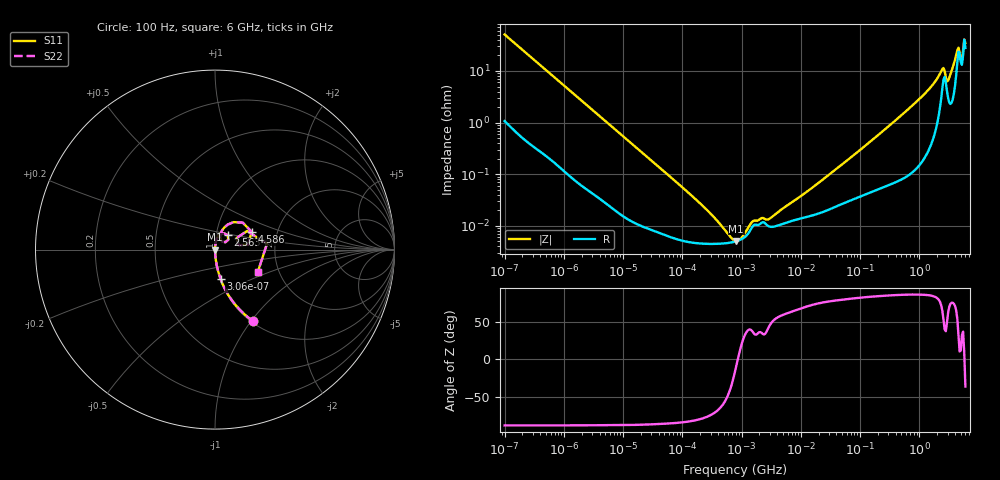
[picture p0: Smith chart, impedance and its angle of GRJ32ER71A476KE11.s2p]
!Murata Part Number: GRJ32ER71A476KE11
!These Parameters are Measured in Series Mode Connection
!Data Generated on Jun 19, 2026
!  o--ll--o
!Port1  Port2
!  o------o
!Operation Temp=25[degC], DC Bias Voltage=0[V]
!Freq. Start=100[Hz] Stop=6[GHz] 401[Steps]
# Hz S RI R 50
!Freq.(Hz) S11(Real) S11(Imag) S21(Real) S21(Imag) S12(Real) S12(Imag) S22(Real) S22(Imag)
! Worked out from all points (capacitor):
!   401 points, 100 Hz to 6 GHz, reference 50 ohm
!   read as one part in series: C = 31 uF near 109 Hz
!   lowest |Z| = 5.06 mohm at 810.1 kHz (marker M1)
!   series resonance near 863.7 kHz, so ESL is about 1.1 nH
!   S11 on the Smith chart (normalised r, x): 100 Hz: 1.02, -1.02; 306 Hz: 1.01, -0.34; 2.563 GHz: 1.14, +0.18; 4.586 GHz: 1.48, +0.31; 6 GHz: 1.56, -0.42
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100  0.2116 -0.3981  0.7884 0.3981  0.7884 0.3981  0.2116 -0.3981
306  0.0308 -0.163  0.9692 0.163  0.9692 0.163  0.0308 -0.163
2008  0.00129 -0.0264  0.9987 0.0264  0.9987 0.0264  0.00129 -0.0264
40335  7.49e-05 -0.00137  0.9999 0.00137  0.9999 0.00137  7.49e-05 -0.00137
184852  4.58e-05 -0.000291  1 0.000291  1 0.000291  4.58e-05 -0.000291
432798  4.49e-05 -9.84e-05  1 9.84e-05  1 9.84e-05  4.49e-05 -9.84e-05
774597  4.92e-05 -1.46e-05  1 1.46e-05  1 1.46e-05  4.92e-05 -1.46e-05
810067  4.99e-05 -8.6e-06  1 8.6e-06  1 8.6e-06  4.99e-05 -8.6e-06
1267578  6.87e-05 5.51e-05  0.9999 -5.51e-05  0.9999 -5.51e-05  6.87e-05 5.51e-05
2169299  0.000114 8.22e-05  0.9999 -8.22e-05  0.9999 -8.22e-05  0.000114 8.22e-05
2967816  9.64e-05 9.74e-05  0.9999 -9.74e-05  0.9999 -9.74e-05  9.64e-05 9.74e-05
1.555665e7  0.000158 0.000522  0.9998 -0.000522  0.9998 -0.000522  0.000158 0.000522
3.124326e8  0.000696 0.00871  0.9993 -0.00871  0.9993 -0.00871  0.000696 0.00871
1.094528e9  0.00268 0.0315  0.9973 -0.0315  0.9973 -0.0315  0.00268 0.0315
2.34314e9  0.037 0.0887  0.963 -0.0887  0.963 -0.0887  0.037 0.0887
2.562649e9  0.0706 0.0797  0.9294 -0.0797  0.9294 -0.0797  0.0706 0.0797
3.065283e9  0.032 0.0543  0.968 -0.0543  0.968 -0.0543  0.032 0.0543
3.666503e9  0.0391 0.1064  0.9609 -0.1064  0.9609 -0.1064  0.0391 0.1064
4.193612e9  0.1026 0.1531  0.8974 -0.1531  0.8974 -0.1531  0.1026 0.1531
4.586474e9  0.2045 0.0991  0.7955 -0.0991  0.7955 -0.0991  0.2045 0.0991
5.245841e9  0.1213 0.0657  0.8787 -0.0657  0.8787 -0.0657  0.1213 0.0657
6e9  0.2388 -0.1234  0.7612 0.1234  0.7612 0.1234  0.2388 -0.1234
